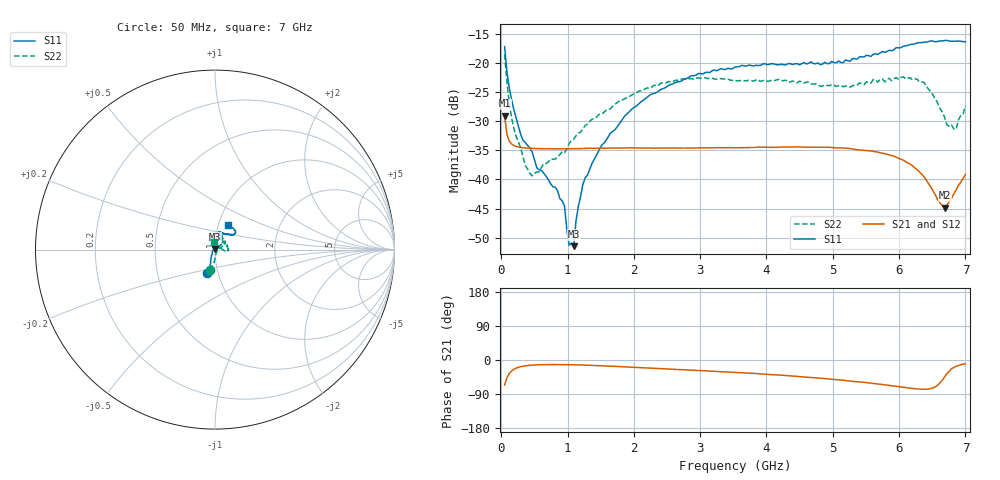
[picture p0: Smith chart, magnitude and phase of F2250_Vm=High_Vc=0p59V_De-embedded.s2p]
! Integrated Device Technology
! Corporate Headquarters
! 6024 Silver Creek Valley Road
! San Jose, CA 95138  USA
! Phone:  1-408-284-8200
! Toll Free:  1-800-223-1366
! Webpage:  http://www.idt.com/
! Timing and RF Division
! 515 Groton Road, Suite 102
! Westford, MA 01886-6024
! Device:  F2250
! Description: Voltage Variable RF Attenuator
! Frequency:  50.0 -  6000.00 MHz
! Package:  3x3 mm Thin QFN Plastic Package: 16 pin
! Ports:  2 RF, 3 DC
!  Pin  1  = GND
!  Pin  2  = NC
!  Pin  3  = RF1  = Port 1
!  Pin  4  = NC
!  Pin  5  = GND
!  Pin  6  = GND
!  Pin  7  = GND
!  Pin  8  = GND
!  Pin  9  = NC
!  Pin 10  = RF2  = Port 2
!  Pin 11  = NC
!  Pin 12  = GND
!  Pin 13  = GND
!  Pin 14  = VCNTRL
!  Pin 15  = VDD
!  Pin 16  = VMODE
! Vcntrl:  0.590 Volts
! Vmode:  +3.300 Volts
! Vdd:  +3.30  Volts
! Current:  1.276 mA
! Data:  The device was measured on a the F2250 evaluation board which has
!  individual transmission lines to the RF pins.  Data was collected
!  using a calibrated network analyzer.  The evaluation board was
!  de-embedded using a TRL calibration technique.
!  The reference plane is the edge of the package pin.
! Misc:  SN 10
!  Action Tracker AT0258
! Date Measured:  2014-11-26
! Date:  2015-10-15  MJV
! Note:
!  Integrated Device Technology supplies this data as a sample of measured
!  data at the package pin for this product.  Your particular data for this
!  product may vary.
!  Data was taken at 25 degrees C.
!  Integrated Device Technology reserves the right to change this data at anytime.
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# GHz S dB R 50
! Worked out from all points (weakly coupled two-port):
!   201 points, 50 MHz to 7 GHz, reference 50 ohm
!   highest |S21| = -29.05 dB at 50 MHz (marker M1); lowest = -44.9 dB at 6.687 GHz (marker M2)
!   lowest |S11| = -51.5 dB at 1.093 GHz (marker M3), VSWR 1.01, Z = 50 + j0.266 ohm
!   |S11| at or under -10 dB: start of sweep to end of sweep
!   |S22| runs from -39.4 to -18.5 dB; largest |S21 - S12| = 5e-05
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0.05  -17.17 -108.4  -29.05 -66.0  -29.05 -66.0  -18.51 -104.2
0.08475  -21.46 -107.2  -32.25 -47.1  -32.25 -47.1  -23.30 -93.2
0.1195  -24.21 -111.7  -33.39 -35.9  -33.39 -35.9  -26.79 -89.6
0.189  -28.00 -119.7  -34.16 -24.6  -34.17 -24.6  -31.21 -81.9
0.328  -33.28 -133.6  -34.56 -16.3  -34.55 -16.3  -36.15 -51.4
0.43225  -34.60 -144.9  -34.64 -13.9  -34.64 -13.9  -38.97 -25.3
0.5365  -38.01 -154.2  -34.68 -12.8  -34.68 -12.8  -38.71 -13.8
0.8145  -41.31 170.1  -34.73 -12.0  -34.73 -12.0  -36.48 10.1
0.9535  -44.56 171.4  -34.74 -12.2  -34.74 -12.3  -35.40 14.3
1.023  -51.30 138.9  -34.73 -12.4  -34.73 -12.4  -33.84 15.5
1.0925  -51.47 85.8  -34.72 -12.6  -34.72 -12.6  -33.07 17.7
1.12725  -47.11 58.6  -34.71 -12.8  -34.71 -12.8  -32.49 15.9
1.2315  -40.78 39.3  -34.68 -13.3  -34.68 -13.3  -31.29 14.4
1.6485  -32.00 40.7  -34.61 -16.3  -34.62 -16.3  -27.80 23.3
2.37825  -24.75 46.4  -34.60 -22.6  -34.60 -22.6  -23.73 32.2
3.525  -20.67 71.6  -34.56 -32.8  -34.56 -32.9  -22.96 59.5
4.7065  -20.07 71.9  -34.44 -46.5  -34.45 -46.5  -23.59 61.9
5.85325  -17.80 40.5  -35.79 -67.1  -35.78 -67.1  -22.62 10.6
6.3745  -16.41 40.9  -39.52 -77.4  -39.52 -77.4  -23.29 -5.9
6.68725  -16.12 47.8  -44.85 -44.3  -44.85 -44.1  -29.34 15.3
6.861  -16.23 54.4  -41.81 -16.4  -41.78 -16.4  -31.35 60.1
7  -16.33 62.4  -39.14 -10.2  -39.11 -10.3  -27.31 95.2
